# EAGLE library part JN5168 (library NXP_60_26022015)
Short Description AAL Eindhoven MK
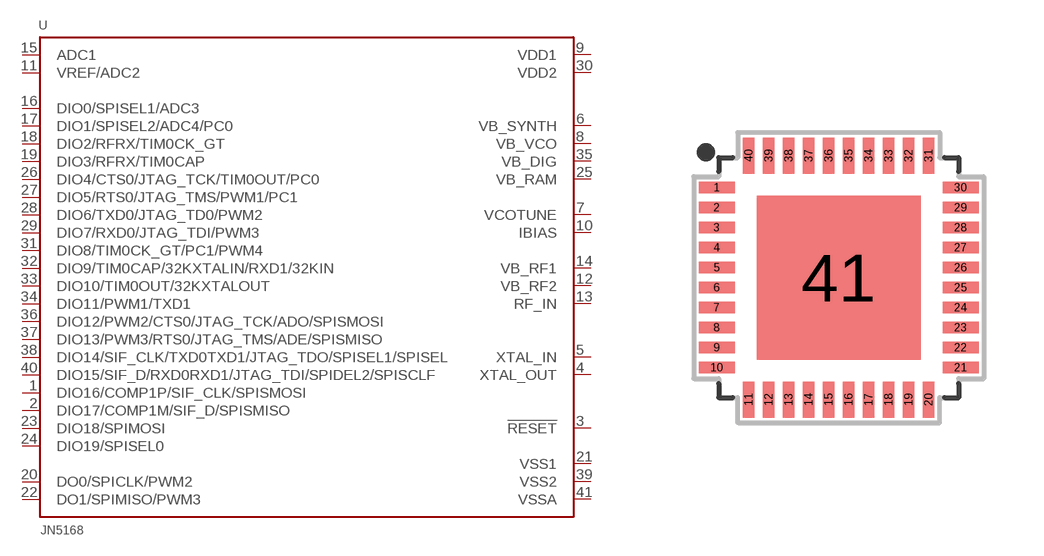
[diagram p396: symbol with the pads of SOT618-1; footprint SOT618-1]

Designator prefix U

## JN5168  [SOT618-1]
1  DIO16/COMP1P/SIF_CLK/SPISMOSI
2  DIO17/COMP1M/SIF_D/SPISMISO
3  !RESET
4  XTAL_OUT
5  XTAL_IN
6  VB_SYNTH
7  VCOTUNE
8  VB_VCO
9  VDD1
10  IBIAS
11  VREF/ADC2
12  VB_RF2
13  RF_IN
14  VB_RF1
15  ADC1
16  DIO0/SPISEL1/ADC3
17  DIO1/SPISEL2/ADC4/PC0
18  DIO2/RFRX/TIM0CK_GT
19  DIO3/RFRX/TIM0CAP
20  DO0/SPICLK/PWM2
21  VSS1
22  DO1/SPIMISO/PWM3
23  DIO18/SPIMOSI
24  DIO19/SPISEL0
25  VB_RAM
26  DIO4/CTS0/JTAG_TCK/TIM0OUT/PC0
27  DIO5/RTS0/JTAG_TMS/PWM1/PC1
28  DIO6/TXD0/JTAG_TD0/PWM2
29  DIO7/RXD0/JTAG_TDI/PWM3
30  VDD2
31  DIO8/TIM0CK_GT/PC1/PWM4
32  DIO9/TIM0CAP/32KXTALIN/RXD1/32KIN
33  DIO10/TIM0OUT/32KXTALOUT
34  DIO11/PWM1/TXD1
35  VB_DIG
36  DIO12/PWM2/CTS0/JTAG_TCK/ADO/SPISMOSI
37  DIO13/PWM3/RTS0/JTAG_TMS/ADE/SPISMISO
38  DIO14/SIF_CLK/TXD0TXD1/JTAG_TDO/SPISEL1/SPISEL
39  VSS2
40  DIO15/SIF_D/RXD0RXD1/JTAG_TDI/SPIDEL2/SPISCLF
41  VSSA

## Footprint SOT618-1 (pad centres in mm)
SOT618-1 HVQFN40: plastic thermal enhanced very thin quad flat package; no leads; 40 terminals; body 6 x 6 x 0.85 mm JEDEC: MO-220 IEC: --
smd 0.9 x 0.29: 1 -3.05,2.25; 2 -3.05,1.75; 3 -3.05,1.25; 4 -3.05,0.75; 5 -3.05,0.25; 6 -3.05,-0.25; 7 -3.05,-0.75; 8 -3.05,-1.25; 9 -3.05,-1.75; 10 -3.05,-2.25; 21 3.05,-2.25; 22 3.05,-1.75; 23 3.05,-1.25; 24 3.05,-0.75; 25 3.05,-0.25; 26 3.05,0.25; 27 3.05,0.75; 28 3.05,1.25; 29 3.05,1.75; 30 3.05,2.25
smd 0.29 x 0.9: 11 -2.25,-3.05; 12 -1.75,-3.05; 13 -1.25,-3.05; 14 -0.75,-3.05; 15 -0.25,-3.05; 16 0.25,-3.05; 17 0.75,-3.05; 18 1.25,-3.05; 19 1.75,-3.05; 20 2.25,-3.05; 31 2.25,3.05; 32 1.75,3.05; 33 1.25,3.05; 34 0.75,3.05; 35 0.25,3.05; 36 -0.25,3.05; 37 -0.75,3.05; 38 -1.25,3.05; 39 -1.75,3.05; 40 -2.25,3.05
smd 4.1 x 4.1: 41 0,0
